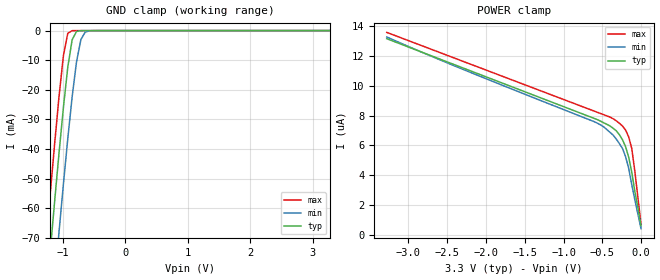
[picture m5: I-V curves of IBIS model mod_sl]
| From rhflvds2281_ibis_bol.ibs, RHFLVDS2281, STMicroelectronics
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|   Model mod_sl
[Model]   mod_sl
Model_type Input
Vinl   =   0.800V
Vinh   =   2.000V
C_comp   0.243pF   0.232pF   0.255pF
[Temperature Range]   25.0000   0.1250k   -55.0000
[Voltage Range]   3.3000V   3.0000V   3.6000V
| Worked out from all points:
|   GND clamp passes 1 mA (typ) near -0.80 V on its own axis
[GND_clamp]
|Voltage   I(typ)   I(min)   I(max)
-3.3V     -613.2mA   -637.8mA   -596mA
-1.27V    -91.44mA   -118.4mA   -71.97mA
-1.2V     -74.37mA   -101.3mA   -54.85mA
-1.13V    -57.62mA   -84.47mA   -38.17mA
-1.06V    -41.37mA   -67.96mA   -22.32mA
-990mV    -26mA      -51.9mA    -8.517mA
-920mV    -12.42mA   -36.55mA   -897uA
-850mV    -3.1mA     -22.41mA   -24.73uA
-780mV    -288uA     -10.57mA   -2.037uA
-710mV    -19.39uA   -3.045mA   -1.412uA
-570mV    -1.205uA   -64.81uA   -1.125uA
3.28V     6.558uA    6.923uA    6.473uA
[POWER_clamp]
|Voltage   I(typ)   I(min)   I(max)
-3.28V    13.16uA    13.27uA    13.58uA
-2.16V    10.92uA    10.81uA    11.37uA
-600mV    7.798uA    7.58uA     8.289uA
-480mV    7.508uA    7.234uA    8.052uA
-360mV    7.148uA    6.687uA    7.785uA
-320mV    6.978uA    6.425uA    7.646uA
-240mV    6.378uA    5.801uA    7.298uA
-200mV    5.918uA    5.257uA    7.029uA
-160mV    5.218uA    4.47uA     6.58uA
-120mV    4.198uA    3.371uA    5.801uA
-80mV     2.918uA    2.344uA    4.263uA
0V        598nA      408.3nA    704.6nA
